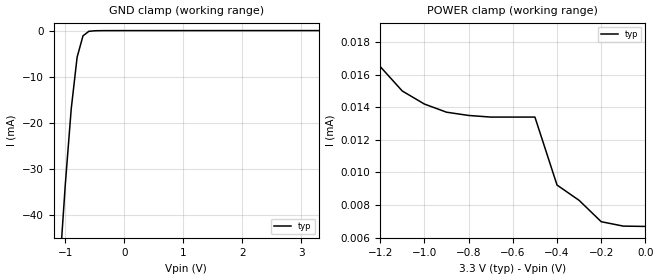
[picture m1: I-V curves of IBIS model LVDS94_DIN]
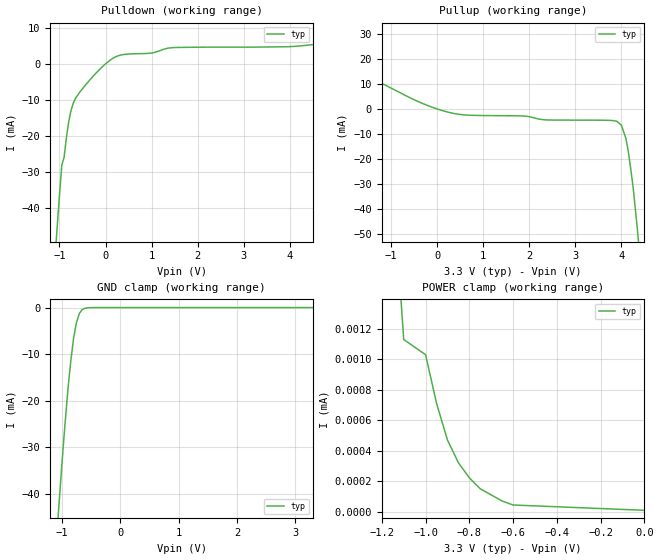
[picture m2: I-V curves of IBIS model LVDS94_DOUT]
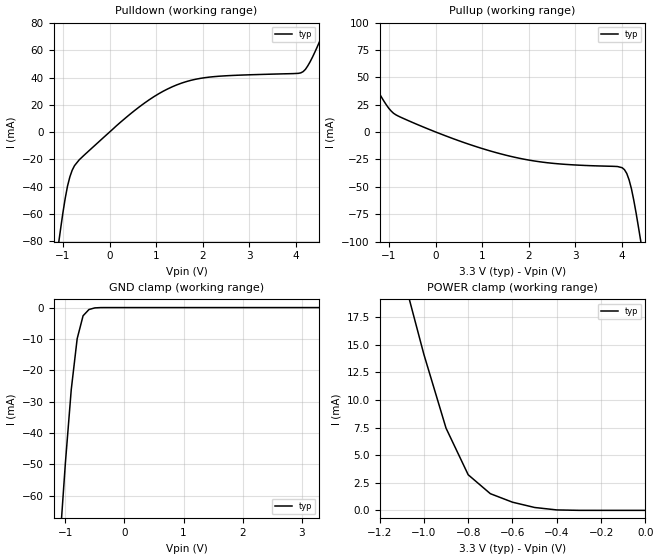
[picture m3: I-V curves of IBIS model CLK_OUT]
|   Texas Instruments Incorporated
|   Data Transmissions Products
|   IBIS Model for SN75LVDS94
|   48DGG Package
[IBIS Ver]   2.1
[Comment char]   |_char
[File name]   65lvds94.ibs
[File Rev]   2.0
[Date]   21Feb97
[Source]   File originated at Texas Instruments Incorporated.
   Data Transmission Products Group. All data based on
   Empirical Measurements(Bench).
[Notes]   File created by Thomas Fisher - Ammended to N-Link 5May99
[Disclaimer]
|(C) Copyright Texas Instruments Incorporated 1997
|   All rights reserved
|  Texas Instruments Incorporated hereby grants the user of this IBIS
|model a non-exclusive, nontransferable license to use this IBIS model
|under the following terms.  Before using this IBIS model, the user
|should read this license.  If the user does not accept these terms,
|the IBIS model should be returned to Texas Instruments within 30 days.
|  The user is granted this license only to use the IBIS model and
|is not granted rights to sell, load, rent, lease or license the IBIS
|model in whole or in part, or in modified form to anyone other than
|user.  User may modify the IBIS model to suit its specific applications
|but rights to derivative works and such modifications shall belong to
|Texas Instruments.
|  This IBIS model is provided on an "AS IS" basis and Texas Instruments
|makes absolutely no warranty with respect to the information contained
|herein.  TEXAS INSTRUMENTS DISCLAIMS AND CUSTOMER WAIVES ALL WARRANTIES,
|EXPRESS OR IMPLIED, INCLUDING WARRANTIES OF MERCHANTABILITY OR FITNESS
|FOR A PARTICULAR PURPOSE. The entire risk as to quality and performance
|is with the Customer. ACCORDINGLY, IN NO EVENT SHALL THE COMPANY BE LIABLE
|FOR ANY DAMAGES, WHETHER IN CONTRACT OR TORT,INCLUDING ANY LOST PROFITS
|OR OTHER INCIDENTAL, CONSEQUENTIAL, EXEMPLARY, OR PUNITIVE DAMAGES ARISING
|OUT OF THE USE OR APPLICATION OF THE IBIS model provided in this package.
|Further, Texas Instruments reserves the right to discontinue or make changes
|without notice to any product herein to improve reliability, function, or
|design. Texas Instruments does not convey any license under patent rights
|or any other intellectual property rights, including those of third parties.
|Contact Texas Instruments at ATTN:DATA TRANSMISSIONS
|Thomas Fisher  8505 Forest Lane, M/S 8710, Dallas, TX 75243-4136
|IBIS Open Forum disclaims all warranties. See DISCLAIM.TXT
|in vhdl.org:/pub/IBIS/models for the full disclaimer.
[Copyright]   Copyright 1997, Texas Instruments, All Rights Reserved
[Component]   SN75LVDS94DGG
[Manufacturer]  Texas Instruments Incorporated
[Package]
|   typ   min   max
R_pkg   0.036   0.022   0.041
L_pkg   2.128nH   2.045nH   2.336nH
C_pkg   0.357pF   0.310pF   0.394pF
[Pin]   signal_name   model_name   R_pin   L_pin   C_pin
1   D22   LVDS94_DOUT   0.038   6.533n   0.795p
2   D23   LVDS94_DOUT   0.038   5.957n   0.824p
3   D24   LVDS94_DOUT   0.039   5.485n   0.725p
4   GND   GND   0.040   5.037n   0.634p
5   D25   LVDS94_DOUT   0.040   4.575n   0.508p
6   D26   LVDS94_DOUT   0.039   4.053n   0.408p
7   D27   LVDS94_DOUT   0.031   3.473n   0.357p
8   LVDSGND   GND   0.028   3.292n   0.367p
9   A0M   LVDS94_DIN   0.027   3.275n   0.353p
10   A0P   LVDS94_DIN   0.027   3.090n   0.318p
11   A1M   LVDS94_DIN   0.027   2.879n   0.277p
12   A1P   LVDS94_DIN   0.027   2.826n   0.286p
13   LVDSVCC   POWER   0.028   2.866n   0.289p
14   LVDSGND   GND   0.028   2.793n   0.288p
15   A2M   LVDS94_DIN   0.028   2.799n   0.288p
16   A2P   LVDS94_DIN   0.026   2.802n   0.288p
17   CLKINM   LVDS94_DIN   0.025   2.746n   0.282p
18   CLKINP   LVDS94_DIN   0.026   2.838n   0.284p
19   A3M   LVDS94_DIN   0.025   2.952n   0.310p
20   A3P   LVDS94_DIN   0.026   3.272n   0.328p
21   LVDSGND   GND   0.028   3.293n   0.373p
22   PLLGND   GND   0.031   3.478n   0.318p
23   PLLVCC   POWER   0.039   4.108n   0.359p
24   PLLGND   GND   0.040   4.592n   0.524p
25   SHTDN   SHTDN_DIN   0.040   5.061n   0.652p
26   CLKOUT   CLK_OUT   0.038   5.507n   0.747p
27   D0   LVDS94_DOUT   0.038   6.003n   0.848p
28   GND   GND   0.036   6.519n   0.769p
29   D1   LVDS94_DOUT   0.036   6.531n   0.769p
30   D2   LVDS94_DOUT   0.038   5.994n   0.847p
31   VCC   POWER   0.038   5.511n   0.747p
32   D3   LVDS94_DOUT   0.040   5.067n   0.653p
33   D4   LVDS94_DOUT   0.040   4.606n   0.525p
34   D5   LVDS94_DOUT   0.040   4.110n   0.423p
35   D6   LVDS94_DOUT   0.030   3.477n   0.366p
36   GND   GND   0.026   3.289n   0.323p
37   D7   LVDS94_DOUT   0.025   2.848n   0.261p
38   D8   LVDS94_DOUT   0.024   2.943n   0.312p
39   D9   LVDS94_DOUT   0.026   2.841n   0.285p
40   VCC   POWER   0.026   2.773n   0.284p
41   D10   LVDS94_DOUT   0.027   2.834n   0.289p
42   D11   LVDS94_DOUT   0.028   2.803n   0.287p
43   D12   LVDS94_DOUT   0.028   2.817n   0.288p
44   GND   GND   0.027   2.836n   0.291p
45   D13   LVDS94_DOUT   0.027   2.824n   0.287p
46   D14   LVDS94_DOUT   0.027   3.242n   0.375p
47   D15   LVDS94_DOUT   0.027   3.000n   0.312p
48   VCC   POWER   0.027   3.298n   0.330p
49   D16   LVDS94_DOUT   0.029   3.305n   0.375p
50   D17   LVDS94_DOUT   0.031   3.858n   0.441p
51   D18   LVDS94_DOUT   0.040   4.131n   0.397p
52   GND   GND   0.041   4.664n   0.481p
53   D19   LVDS94_DOUT   0.040   5.089n   0.654p
54   D20   LVDS94_DOUT   0.040   5.566n   0.753p
55   D21   LVDS94_DOUT   0.038   6.009n   0.854p
56   VCC   POWER   0.039   6.620n   0.810p
[Diff_pin]   inv_pin   vdiff   tdelay_typ   tdelay_min   tdelay_max
| The 'AXP' pin is Diff_pin and the 'AXM' pin is the inv_pin
| The 'CLKINP' pin is Diff_pin and the 'CLKINM' pin is the inv_pin
12   11   100mV   0 0 0   | Vth  +/-100mV
10   9   100mV   0 0 0
16   15   100mV   0 0 0
20   19   100mV   0 0 0
18   17   100mV   0 0 0
| Models and submodels in the file (4): LVDS94_DIN (Input), SHTDN_DIN (Input), LVDS94_DOUT (3-state), CLK_OUT (3-state)
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|   Driver Input  MODEL
[Model]   LVDS94_DIN
Model_type   Input
|Signals   D0,D1,D2,D3,D4,D5,D6,D7,D8,D9,D10,D11,D12,D13,D14,D15,D16,
|   D17,D18,D19,D20,SHTDN,CLKIN
Vinh = 2.0
Vinl = 0.8
|   typ   min   max
C_comp   1.0pF   NA   NA
|   typ   min   max
[Temperature Range]   25.0   NA   NA
[Voltage range]   3.3V   3.0V   3.6V
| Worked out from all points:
|   GND clamp passes 1 mA (typ) near -0.69 V on its own axis
[Power_clamp]
| Note that the[POWER_clamp]voltage table is referenced to Vcc
| and is calculated using Vtable=Vcc - Vmeasured.
|   Voltage   I(typ)   I(min)   I(max)
-3.3V     780uA      NA         NA
-1.3V     19.1uA     NA         NA
-1.2V     16.5uA     NA         NA
-1.1V     15uA       NA         NA
-1V       14.2uA     NA         NA
-900mV    13.7uA     NA         NA
-800mV    13.5uA     NA         NA
-500mV    13.4uA     NA         NA
-400mV    9.23uA     NA         NA
-300mV    8.29uA     NA         NA
-200mV    6.98uA     NA         NA
0V        6.69uA     NA         NA
[GND_clamp]
|   Voltage   I(typ)   I(min)   I(max)
-3.3V     -485.8mA   NA         NA
-1.1V     -52.3mA    NA         NA
-1V       -33.38mA   NA         NA
-900mV    -17.03mA   NA         NA
-800mV    -5.78mA    NA         NA
-700mV    -1.13mA    NA         NA
-600mV    -150uA     NA         NA
-300mV    -2.96uA    NA         NA
3.3V      6.69uA     NA         NA
|   Driver Output  MODEL
[Model]   LVDS94_DOUT
Model_type   3-state
| Signals   Y0P,Y0M,Y1P,Y1M,Y2P,Y2M,CLKOUTP,CLKOUTM
Vmeas = 1.2V   |Reference voltage for timing measurements
Cref = 5pF   |Timing specification test load capacitance value
Rref = 50   |Note: 50 Ohm load; single ended configuration
Vref = 1.18V   |Timing specification test load voltage
| variable   typ   min   max
C_comp   1.0pF   NA   NA
|   typ   min   max
[Temperature Range]   25.0   NA   NA
[Voltage range]   3.3V   3.0V   3.6V
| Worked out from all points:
|   slope of the pulldown table from 0 to 0.495 V, typ, clamps not added: 182 ohm
|   slope of the pullup table from 0 to 0.495 V, typ, clamps not added: 224 ohm
|   GND clamp passes 1 mA (typ) near -0.69 V on its own axis
[Pulldown]
|   Voltage   I(typ)   I(min)   I(max)
-3.3V     -466.3mA   NA         NA
-1.1V     -54.41mA   NA         NA
-1.05V    -45.42mA   NA         NA
-950mV    -28.23mA   NA         NA
-900mV    -26.02mA   NA         NA
-800mV    -16.18mA   NA         NA
-700mV    -10.96mA   NA         NA
-250mV    -3.21mA    NA         NA
250mV     2.077mA    NA         NA
1.45V     4.458mA    NA         NA
4.15V     4.857mA    NA         NA
6.6V      9.522mA    NA         NA
[Pullup]
|   Voltage   I(typ)   I(min)   I(max)
| Note that the[Pullup]voltage table is referenced to Vcc
| and is calculated using Vtable=Vcc - Vmeasured.
-3.3V     32.52mA    NA         NA
-1.3V     11.15mA    NA         NA
200mV     -1.15mA    NA         NA
2.4V      -4.46mA    NA         NA
3.9V      -4.96mA    NA         NA
4V        -6.51mA    NA         NA
4.1V      -11.9mA    NA         NA
4.15V     -17.01mA   NA         NA
4.25V     -30.57mA   NA         NA
4.35V     -48.72mA   NA         NA
4.4V      -58.4mA    NA         NA
6.6V      -501.5mA   NA         NA
[GND_clamp]
|   Voltage   I(typ)   I(min)   I(max)
| Outputs in Tri-state.
-3.3V     -462.7mA   NA         NA
-1.1V     -51.07mA   NA         NA
-1.05V    -42.1mA    NA         NA
-950mV    -25.35mA   NA         NA
-900mV    -17.89mA   NA         NA
-850mV    -11.64mA   NA         NA
-800mV    -6.53mA    NA         NA
-750mV    -3.14mA    NA         NA
-700mV    -1.23mA    NA         NA
-650mV    -410uA     NA         NA
-450mV    -2.68uA    NA         NA
3.3V      16.9nA     NA         NA
[POWER_clamp]
|   Voltage   I(typ)   I(min)   I(max)
| Note that the [POWER_clamp] voltage table is referenced to Vcc
| and is calculated using Vtable = Vcc - Vmeasured.
| Outputs in Tri-state.
-3.3V     729uA      NA         NA
-1.15V    2.18uA     NA         NA
-1.1V     1.13uA     NA         NA
-1V       1.03uA     NA         NA
-950mV    712nA      NA         NA
-900mV    471nA      NA         NA
-850mV    322nA      NA         NA
-800mV    223nA      NA         NA
-750mV    151nA      NA         NA
-650mV    70.7nA     NA         NA
-600mV    45nA       NA         NA
0V        10.2nA     NA         NA
[Ramp]
| Note: Ramp rate measured on single-ended Driver Output.
|   typ   min   max
dV/dt_r   0.200/258ps   NA   NA
dV/dt_f   0.200/250ps   NA   NA
R_load = 100ohm | Note: These are single ended driver measurements
|   with 100ohm line-to-line termination and 4.5pF
|   line-to-ground capacitive load
|   Receiver Clock Output  MODEL
[Model]   CLK_OUT
Model_type   3-state
| Signals   CLKOUT
Vmeas = 1.5V   |Reference voltage for timing measurements
Cref = 8pF   |Timing specification test load capacitance value
Vref = 0   |Timing specification test load voltage; GND
| variable   typ   min   max
C_comp   1.0pF   NA   NA
|   typ   min   max
[Temperature Range]   25.0   NA   NA
[Voltage range]   3.3V   3.0V   3.6V
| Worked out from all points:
|   slope of the pulldown table from 0 to 0.495 V, typ, clamps not added: 33.8 ohm
|   slope of the pullup table from 0 to 0.495 V, typ, clamps not added: 62.3 ohm
|   GND clamp passes 1 mA (typ) near -0.62 V on its own axis
|   POWER clamp passes 1 mA (typ) near -0.63 V on its own axis
[Pulldown]
|   Voltage   I(typ)   I(min)   I(max)
-3.3V     -629.8mA   NA         NA
-1.1V     -83.77mA   NA         NA
-1.05V    -71.36mA   NA         NA
-900mV    -39.59mA   NA         NA
-750mV    -24.61mA   NA         NA
450mV     13.38mA    NA         NA
1.35V     33.29mA    NA         NA
2.15V     40.35mA    NA         NA
4.1V      43.42mA    NA         NA
4.25V     48.53mA    NA         NA
4.5V      66.15mA    NA         NA
6.6V      231.7mA    NA         NA
[Pullup]
|   Voltage   I(typ)   I(min)   I(max)
| Note that the[Pullup]voltage table is referenced to Vcc
| and is calculated using Vtable=Vcc - Vmeasured.
-3.3V     188.7mA    NA         NA
-1.2V     34.95mA    NA         NA
-900mV    17.2mA     NA         NA
-300mV    5.322mA    NA         NA
800mV     -12.3mA    NA         NA
1.8V      -23.95mA   NA         NA
4V        -32.53mA   NA         NA
4.1V      -37.83mA   NA         NA
4.15V     -43.73mA   NA         NA
4.25V     -62.28mA   NA         NA
4.4V      -99.75mA   NA         NA
6.6V      -670.4mA   NA         NA
[GND_clamp]
|   Voltage   I(typ)   I(min)   I(max)
| Outputs in Tri-state.
-3.3V     -740mA     NA         NA
-1.1V     -76.92mA   NA         NA
-1V       -49.78mA   NA         NA
-900mV    -26.17mA   NA         NA
-800mV    -9.95mA    NA         NA
-700mV    -2.62mA    NA         NA
-600mV    -620uA     NA         NA
-500mV    -100uA     NA         NA
-400mV    -5.98uA    NA         NA
3.3V      350pA      NA         NA
[POWER_clamp]
|   Voltage   I(typ)   I(min)   I(max)
| Note that the [POWER_clamp] voltage table is referenced to Vcc
| and is calculated using Vtable = Vcc - Vmeasured.
| Outputs in Tri-state.
-3.3V     208.5mA    NA         NA
-1.1V     21.72mA    NA         NA
-1V       14.13mA    NA         NA
-900mV    7.445mA    NA         NA
-800mV    3.224mA    NA         NA
-700mV    1.51mA     NA         NA
-600mV    739uA      NA         NA
-500mV    260uA      NA         NA
-400mV    38.9uA     NA         NA
0V        -9.18nA    NA         NA
[Ramp]
|   typ   min   max
dV/dt_r   1.903v/533ps   NA   NA
dV/dt_f   1.922v/565ps   NA   NA
R_load = 1000ohm
